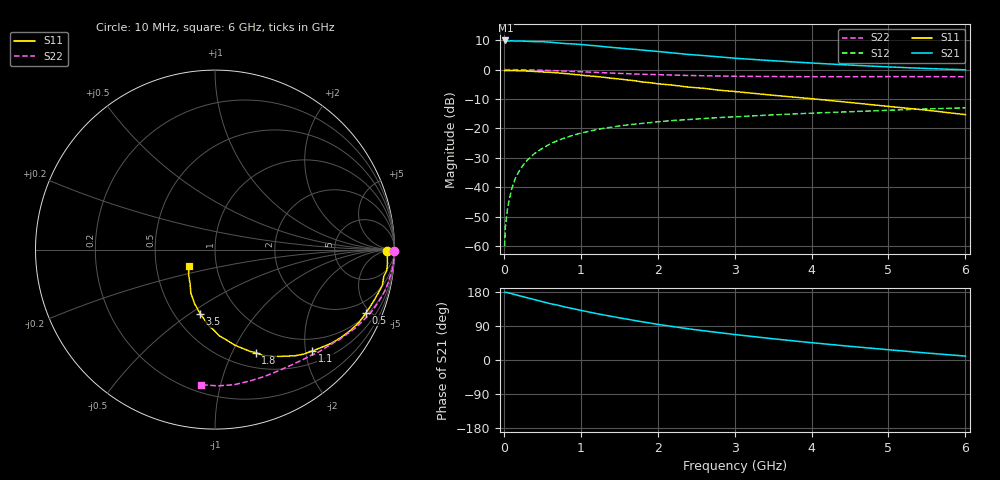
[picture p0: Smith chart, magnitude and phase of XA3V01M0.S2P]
! SIEMENS Discrete & RF Semiconductors
! BFY180
! Si NPN RF Bipolar Junction Transistor in MICRO-X
! VCE = 3 V  IC = 1 mA
! Common Emitter S-Parameters:  May  1997
# GHz  S  MA  R  50
!  f  S11  S21  S12  S22
! GHz  MAG  ANG  MAG  ANG  MAG  ANG  MAG  ANG
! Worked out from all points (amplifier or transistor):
!   36 points, 10 MHz to 6 GHz, reference 50 ohm
!   highest |S21| = 9.9 dB at 20 MHz (marker M1)
!   |S21| within 3 dB of that: start of sweep to 1.697 GHz
!   unconditionally stable (mu >= 1): 3.847 GHz to end of sweep
!   at 250 MHz: K = 0.08, MSG = 21.1 dB, |S12| = -32.5 dB
!   at 1.4 GHz: K = 0.51, MSG = 13.6 dB, |S12| = -19.6 dB
!   at 6 GHz: K = 1.06, MAG = 5.0 dB, |S12| = -13.0 dB
!   S11 on the Smith chart (normalised r, x): 10 MHz: 48, -10; 500 MHz: 1.13, -4.75; 1.1 GHz: 0.73, -2.14; 1.8 GHz: 0.67, -1.24; 3.5 GHz: 0.67, -0.55; 6 GHz: 0.73, -0.14
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0.01  0.9609 -0.5  3.078 179.5  0.001 80.4  0.9972 -0.3
0.02  0.9674 -0.9  3.131 178.7  0.0021 87.4  0.9999 -0.5
0.05  0.9602 -1.9  3.051 177.6  0.0046 87.6  0.9974 -1.4
0.1  0.9642 -4.7  3.091 175.0  0.0092 88.9  0.9978 -2.7
0.15  0.9637 -7.0  3.055 172.4  0.0144 84.8  0.9979 -4.0
0.3  0.9464 -13.7  3.032 164.4  0.0285 80.7  0.9886 -8.0
0.5  0.9129 -22.6  2.983 154.0  0.0459 74.3  0.9762 -13.2
0.6  0.8998 -26.6  2.927 148.7  0.0545 71.6  0.9653 -15.6
0.8  0.8577 -34.6  2.772 139.6  0.0695 65.8  0.9445 -20.3
1  0.8073 -42.3  2.674 131.1  0.0834 60.7  0.9205 -24.7
1.1  0.7833 -46.1  2.6 126.9  0.0891 58.2  0.9086 -26.8
1.2  0.7635 -49.7  2.535 122.7  0.0954 55.8  0.8976 -28.8
1.5  0.6931 -59.2  2.329 111.3  0.1103 50.2  0.8634 -34.2
1.8  0.6164 -68.5  2.151 100.7  0.1222 45.5  0.8356 -39.1
2  0.5755 -73.9  2.037 94.0  0.13 42.6  0.8212 -42.2
2.2  0.5445 -78.2  1.922 88.2  0.1367 39.8  0.8093 -45.3
2.4  0.5048 -83.2  1.811 82.3  0.1417 37.6  0.7948 -48.0
2.8  0.447 -91.1  1.647 72.2  0.1531 33.8  0.7787 -53.3
3.5  0.3668 -103.0  1.415 56.0  0.1704 27.8  0.7625 -62.1
4.5  0.2764 -119.2  1.195 36.1  0.1927 20.0  0.7573 -75.1
5.5  0.2045 -135.9  1.045 18.4  0.2149 12.2  0.7594 -88.9
6  0.1718 -148.2  0.993 10.3  0.2242 8.1  0.7565 -95.8
